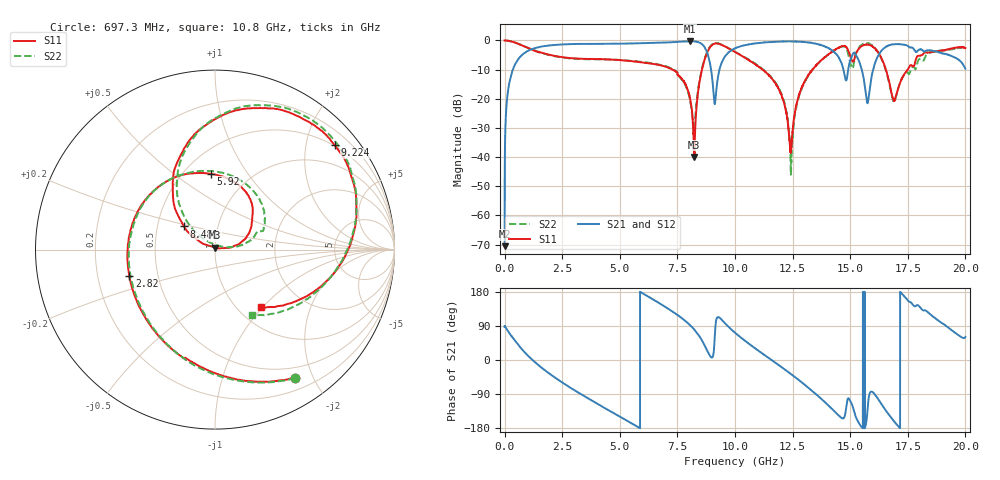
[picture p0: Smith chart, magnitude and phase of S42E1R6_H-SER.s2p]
!{S42E1R6}
!Johanson Technology Inc.
!www.johansontechnology.com
!Test Board Conditions:
!Substrate Type  RO4350B
!Substrate Thickness  50 mil
!Substrate Dk  3.66
!TL Type: GCPW
!TL Trace Width  60 mil
!TL Gap  10 mil
!Electrode orientation  Horizontal
!DUT TOPOLOGY	SERIES
!Mounting Pad LxW  14x55 mil
! Created Wed Nov 25 21:35:21 2020
# khz S ma R 50
! 2 Port Network Data from SP1.SP block
! freq  magS11  angS11  magS21  angS21  magS12  angS12  magS22  angS22
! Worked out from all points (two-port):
!   20001 points, 300 kHz to 20 GHz, reference 50 ohm
!   highest |S21| = -0.28 dB at 8.062 GHz (marker M1); lowest = -70.6 dB at 300 kHz (marker M2)
!   |S21| within 3 dB of the highest: 1.089 GHz to 8.747 GHz (7.658 GHz wide, 156 % of centre); 9.863 GHz to 14.19 GHz (4.331 GHz wide, 36 % of centre)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
!   lowest |S11| = -40.0 dB at 8.236 GHz (marker M3), VSWR 1.02, Z = 50.1 + j0.998 ohm
!   |S11| at or under -10 dB: 7.293 GHz to 8.566 GHz (1.273 GHz wide, 16.1 % of centre); 11.19 GHz to 13.36 GHz (2.17 GHz wide, 17.7 % of centre); 16.55 GHz to 17.5 GHz (948.3 MHz wide, 5.57 % of centre)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
!   |S22| runs from -46.1 to 0.0 dB; largest |S21 - S12| = 0.017
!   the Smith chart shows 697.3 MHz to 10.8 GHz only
!   S11 on the Smith chart (normalised r, x): 697.3 MHz: 0.36, -1.75; 2.82 GHz: 0.34, -0.13; 5.92 GHz: 0.67, +0.69; 8.481 GHz: 0.69, +0.19; 9.224 GHz: 0.48, +2.59; 10.8 GHz: 1.27, -0.97
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300  0.9996 -0.3  0.0002964 87.6  0.0003478 96.6  1 -0.3
157300  0.988 -14.3  0.1451 75.4  0.1465 75.3  0.9875 -14.2
697300  0.8416 -58.0  0.535 32.1  0.5352 32.3  0.8436 -58.0
2820300  0.5004 -162.7  0.8637 -71.8  0.864 -71.7  0.4943 -161.0
3334300  0.486 176.6  0.8718 -90.9  0.8714 -90.9  0.4812 -178.8
5920300  0.4227 92.9  0.8971 178.5  0.8957 178.6  0.4305 85.1
6667300  0.3819 69.3  0.9151 151.6  0.9134 151.6  0.3882 55.9
8062300  0.09465 8.9  0.9683 91.2  0.9652 91.4  0.08819 9.6
8236300  0.01 85.6  0.9614 80.2  0.9606 80.2  0.02886 97.0
8481300  0.2153 143.3  0.9101 60.2  0.9105 60.2  0.229 134.6
9224300  0.8848 41.0  0.1881 112.1  0.1878 112.7  0.9019 42.2
1.00003e7  0.6345 -17.4  0.7334 72.1  0.7317 72.3  0.6372 -17.9
1.07953e7  0.4092 -51.5  0.8807 34.3  0.8851 34.4  0.4193 -60.2
1.19593e7  0.13 -92.2  0.9593 -16.1  0.9591 -16.2  0.135 -117.9
1.24273e7  0.01247 -11.2  0.9619 -37.1  0.9634 -37.3  0.005027 137.1
1.33343e7  0.3034 16.8  0.9059 -80.8  0.908 -80.5  0.3039 0.4
1.43333e7  0.6871 -44.2  0.6182 -136.5  0.6234 -136.4  0.6872 -54.5
1.52453e7  0.5845 -82.2  0.573 -150.3  0.5735 -150.6  0.6023 -74.2
1.57503e7  0.8522 -128.2  0.08421 -133.0  0.08416 -133.7  0.8923 -126.7
1.66673e7  0.213 166.4  0.8224 -143.5  0.8179 -143.6  0.205 155.9
1.83283e7  0.6247 -144.3  0.6729 128.3  0.6738 129.1  0.5783 -141.0
2e7  0.7355 139.3  0.3276 60.7  0.3309 61.7  0.7489 128.6
